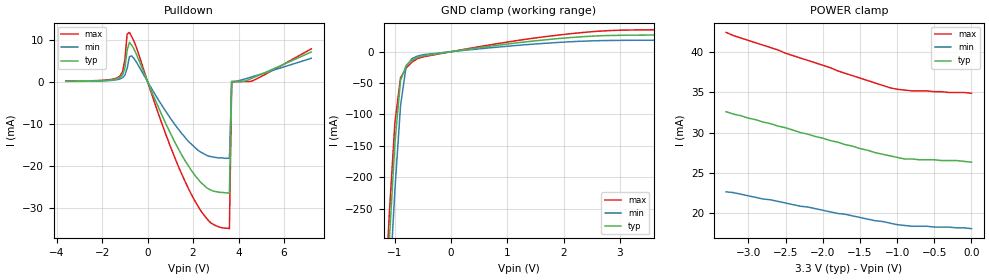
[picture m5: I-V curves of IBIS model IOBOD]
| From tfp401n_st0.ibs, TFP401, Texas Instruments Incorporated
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|   OPEN DRAIN INPUT / OUTPUT  MODEL
[Model]   IOBOD
Model_type   I/O_open_sink
Vinl = 0.8
Vinh = 2.0
| variable   typ   min   max
C_comp   2pF   NA   NA
|   typ   min   max
[Temperature Range]   25.0   70   0
[Voltage range]   3.3V   3.0V   3.6V
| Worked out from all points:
|   GND clamp passes 1 mA (typ) near -0.08 V on its own axis
[GND_clamp]
|Voltage   I(typ)   I(min)   I(max)
-3.6V     -5.15A     -5.23A     -5.11A
-1.2V     -476mA     -561mA     -431mA
-1.1V     -302mA     -384mA     -259mA
-1V       -146mA     -220mA     -113mA
-900mV    -45.9mA    -86mA      -41.7mA
-800mV    -21.9mA    -23.2mA    -26.2mA
-700mV    -13.9mA    -11.3mA    -17mA
-600mV    -9.06mA    -7mA       -11.1mA
600mV     7.59mA     5.39mA     9.53mA
1.9V      20.8mA     14.7mA     26.4mA
2.6V      25.1mA     17.5mA     32.5mA
3.6V      26.5mA     18.3mA     34.9mA
[Power_clamp]
|Note that the [Power_clamp] voltage table is referenced to Vcc
|and is calculated using Vtable=Vcc-Vmeasured.
|Voltage   I(typ)   I(min)   I(max)
-3.3V     32.6mA     22.6mA     42.5mA
-3.2V     32.3mA     22.5mA     42.1mA
-2.6V     30.8mA     21.4mA     40.3mA
-2.5V     30.6mA     21.2mA     39.9mA
-2.3V     30mA       20.8mA     39.3mA
-2.2V     29.8mA     20.7mA     39mA
-1.7V     28.5mA     19.8mA     37.4mA
-1.3V     27.5mA     19mA       36.2mA
-1.1V     27.1mA     18.7mA     35.6mA
-900mV    26.7mA     18.4mA     35.3mA
-200mV    26.5mA     18.1mA     35mA
0V        26.3mA     18mA       34.9mA
[Pulldown]
|Voltage   I(typ)   I(min)   I(max)
-3.6V     99.7uA     73.1uA     120uA
-1.3V     784uA      511uA      1.02mA
-1.1V     1.66mA     952uA      2.4mA
-900mV    7.52mA     3.2mA      11.3mA
-800mV    9.35mA     5.94mA     11.7mA
1V        -12.2mA    -8.66mA    -15.4mA
1.9V      -20.9mA    -14.7mA    -26.5mA
2.8V      -25.8mA    -17.8mA    -33.6mA
3.6V      -26.5mA    -18.2mA    -34.9mA
3.7V      20.4uA     29.5uA     6.05uA
4.6V      830uA      1.16mA     179uA
7.2V      7.04mA     5.55mA     7.78mA
[Ramp]
|   typ   min   max
dV/dt_f   1.96v/500ps   1.86v/800ps   1.84v/300ps
dV/dt_r   1mv/1us   1mv/1us   1mv/1us
R_load = 5K
